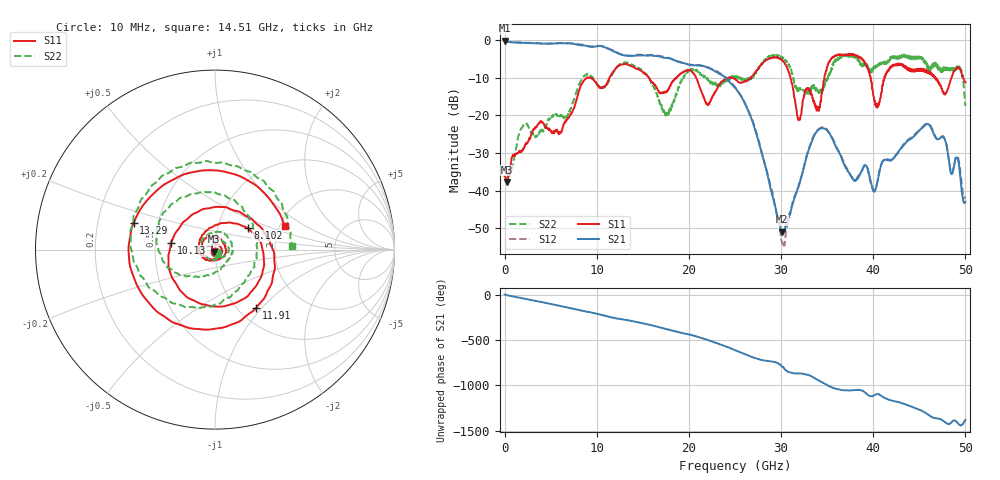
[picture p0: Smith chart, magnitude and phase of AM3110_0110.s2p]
# Hz S DB R 50.0
!freq dBS11 angS11 dBS21 angS21 dBS12 angS12 dBS22 angS22
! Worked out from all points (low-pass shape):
!   1601 points, 10 MHz to 50 GHz, reference 50 ohm
!   highest |S21| = -0.12 dB at 10 MHz (marker M1); lowest = -50.9 dB at 30.13 GHz (marker M2)
!   |S21| within 3 dB of the highest: start of sweep to 11.99 GHz
!   lowest |S11| = -37.7 dB at 228.7 MHz (marker M3), VSWR 1.03, Z = 49.3 - j1.09 ohm
!   |S11| at or under -10 dB: start of sweep to 8.916 GHz; 20.78 GHz to 24.31 GHz (3.526 GHz wide, 15.6 % of centre); 31.02 GHz to 34.7 GHz (3.687 GHz wide, 11.2 % of centre)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
!   |S22| runs from -36.3 to -3.8 dB; largest |S21 - S12| = 0.022
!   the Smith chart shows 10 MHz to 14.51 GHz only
!   S11 on the Smith chart (normalised r, x): 10 MHz: 1.00, -0.03; 8.102 GHz: 1.39, +0.35; 10.13 GHz: 0.60, +0.05; 11.91 GHz: 1.20, -0.93; 13.29 GHz: 0.36, +0.14; 14.51 GHz: 2.13, +0.66
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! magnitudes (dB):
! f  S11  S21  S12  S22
! 10 MHz  -36.2  -0.1  -0.1  -33.6
! 228.7 MHz  -37.7  -0.3  -0.3  -35.9
! 1.978 GHz  -29.0  -0.7  -0.6  -22.9
! 8.102 GHz  -13.2  -1.3  -1.1  -11.7
! 8.352 GHz  -11.7  -1.4  -1.2  -10.5
! 10.13 GHz  -12.1  -1.6  -1.5  -11.9
! 11.91 GHz  -8.0  -3.0  -2.9  -8.3
! 13.29 GHz  -6.4  -4.1  -4.1  -6.0
! 14.51 GHz  -7.7  -4.1  -3.9  -7.3
! 16.69 GHz  -13.5  -4.3  -4.2  -15.6
! 25 GHz  -10.4  -12.7  -12.5  -9.8
! 27.19 GHz  -8.6  -23.8  -23.4  -8.8
! 30.13 GHz  -5.3  -50.9  -54.0  -4.5
! 31.91 GHz  -21.2  -38.9  -38.6  -13.5
! 33.35 GHz  -14.4  -26.9  -26.5  -12.2
! 34.91 GHz  -8.2  -23.8  -23.5  -11.0
! 37.63 GHz  -3.7  -36.4  -36.3  -4.1
! 40.1 GHz  -15.7  -40.2  -40.0  -6.9
! 41.69 GHz  -7.8  -31.9  -31.8  -5.8
! 45.97 GHz  -8.3  -22.4  -22.2  -7.9
! 49.34 GHz  -7.5  -33.9  -32.9  -7.0
! 50 GHz  -11.2  -43.0  -41.6  -17.5
